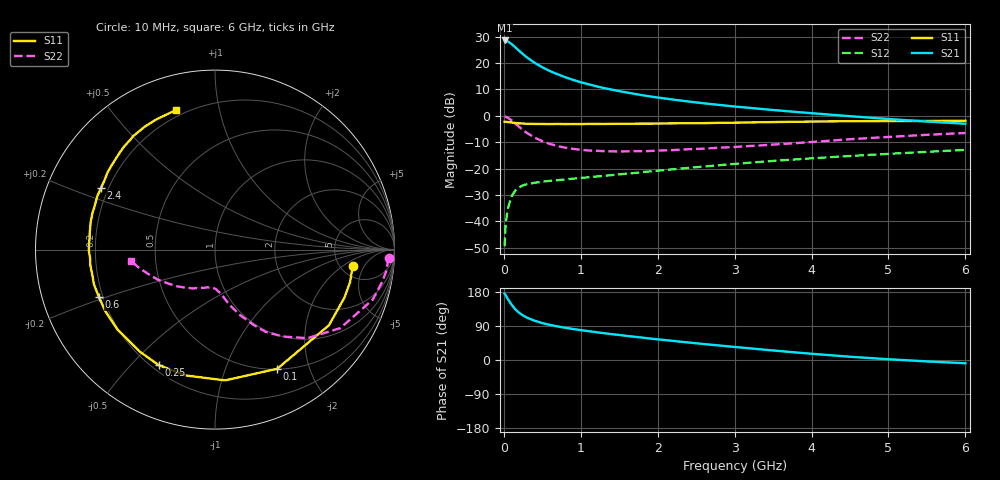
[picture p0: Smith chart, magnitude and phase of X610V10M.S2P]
! SIEMENS Small Signal Semiconductors
! BFP193W
! Si NPN RF Bipolar Junction Transistor in SOT343
! VCE = 10 V  IC = 10 mA
! Common Emitter S-Parameters:  April 1994
# GHz  S  MA  R  50
!  f  S11  S21  S12  S22
! GHz  MAG  ANG  MAG  ANG  MAG  ANG  MAG  ANG
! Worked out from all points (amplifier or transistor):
!   40 points, 10 MHz to 6 GHz, reference 50 ohm
!   highest |S21| = 28.5 dB at 10 MHz (marker M1)
!   |S21| within 3 dB of that: start of sweep to 164.8 MHz
!   unconditionally stable (mu >= 1): 1.389 GHz to 4.621 GHz
!   at 200 MHz: K = 0.22, MSG = 25.8 dB, |S12| = -27.1 dB
!   at 1.5 GHz: K = 1.04, MAG = 14.6 dB, |S12| = -22.2 dB
!   at 6 GHz: K = 0.93, MSG = 4.9 dB, |S12| = -12.9 dB
!   S11 on the Smith chart (normalised r, x): 10 MHz: 6.51, -2.87; 100 MHz: 0.51, -1.53; 250 MHz: 0.23, -0.60; 600 MHz: 0.18, -0.19; 2.4 GHz: 0.17, +0.25; 6 GHz: 0.17, +0.74
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0.01  0.7729 -6.6  26.76 175.0  0.0034 81.4  0.9687 -2.8
0.02  0.774 -13.6  26.75 172.3  0.0072 78.9  0.9612 -7.3
0.03  0.7691 -20.4  26.53 168.8  0.0105 78.7  0.9495 -10.7
0.05  0.762 -33.6  25.75 161.6  0.017 73.4  0.922 -17.6
0.1  0.749 -62.4  22.92 146.2  0.0299 60.6  0.8236 -32.1
0.15  0.7309 -85.6  19.84 133.6  0.0387 50.6  0.713 -43.8
0.2  0.7197 -103.0  16.97 124.4  0.0442 44.3  0.6155 -51.9
0.25  0.7161 -116.0  14.7 117.5  0.0484 39.8  0.5393 -58.3
0.3  0.706 -126.1  12.79 111.8  0.0507 36.8  0.4739 -62.7
0.4  0.7025 -140.5  10.11 103.6  0.054 33.1  0.3871 -69.4
0.5  0.7009 -150.6  8.32 97.4  0.0566 31.9  0.3317 -73.9
0.6  0.6986 -157.8  7.026 92.6  0.0587 31.5  0.2932 -77.5
0.8  0.6978 -168.6  5.371 85.0  0.0626 32.5  0.2491 -82.4
1.1  0.7029 -179.4  3.964 76.1  0.0686 35.2  0.2203 -88.6
1.3  0.7014 174.8  3.364 70.8  0.073 37.0  0.2147 -92.2
1.6  0.7098 167.4  2.765 63.5  0.0804 39.6  0.2128 -97.4
2.2  0.7201 155.4  2.032 50.4  0.0972 43.0  0.2246 -108.6
2.4  0.722 151.5  1.865 46.2  0.1033 43.5  0.2333 -112.0
3.2  0.749 137.7  1.414 30.8  0.1297 43.7  0.2685 -127.5
4.5  0.7891 119.5  0.984 8.6  0.1735 39.7  0.3605 -152.4
5.5  0.7989 110.0  0.78 -3.7  0.208 35.3  0.4369 -166.8
6  0.8067 105.8  0.708 -8.6  0.2267 33.2  0.4735 -172.5
